(* Logix 5000 Rung export; software revision 24.00 *)

TYPE SNAPP_CONTROL_22 :
STRUCT
   Reserved_0_0 : BOOL;
   Trigger : BOOL;
   Reserved_0_2 : BOOL;
   InspectionResultsAck : BOOL;
   ExecuteCommand : BOOL;
   Reserved_0_5 : BOOL;
   Reserved_0_6 : BOOL;
   Reserved_0_7 : BOOL;
   Reserved_Byte1 : SINT;
   Reserved_2_0 : BOOL;
   Reserved_2_1 : BOOL;
   ClearError : BOOL;
   Reserved_2_3 : BOOL;
   Reserved_2_4 : BOOL;
   Reserved_2_5 : BOOL;
   Reserved_2_6 : BOOL;
   Reserved_2_7 : BOOL;
   Reserved_3_0 : BOOL;
   Reserved_3_1 : BOOL;
   Reserved_3_2 : BOOL;
   Reserved_3_3 : BOOL;
   Reserved_3_4 : BOOL;
   Reserved_3_5 : BOOL;
   Reserved_3_6 : BOOL;
   Reserved_3_7 : BOOL;
   CommandID : INT;
   Reserved_Bytes6and7 : INT;
END_STRUCT
END_TYPE

TYPE SNAPP_IN_13 :
STRUCT
   Status : SNAPP_STAT_IN_13;
   InspectionResults : SNAPP_RESULTS_13;
END_STRUCT
END_TYPE

TYPE SNAPP_STAT_IN_13 :
STRUCT
   TriggerReady : BOOL;
   TriggerAck : BOOL;
   Reserved_0_2 : BOOL;
   AcqError : BOOL;
   Reserved_0_4 : BOOL;
   Reserved_0_5 : BOOL;
   Reserved_0_6 : BOOL;
   Online : BOOL;
   Reserved_1_0 : BOOL;
   InspectionCompleted : BOOL;
   Reserved_1_2 : BOOL;
   ResultsValid : BOOL;
   CommandExecuting : BOOL;
   CommandCompleted : BOOL;
   CommandFailed : BOOL;
   Error : BOOL;
   Reserved_2_0 : BOOL;
   Reserved_2_1 : BOOL;
   Reserved_2_2 : BOOL;
   Reserved_2_3 : BOOL;
   InspectionPass : BOOL;
   Reserved_2_5 : BOOL;
   Reserved_2_6 : BOOL;
   Reserved_2_7 : BOOL;
   Reserved_3_0 : BOOL;
   Reserved_3_1 : BOOL;
   Reserved_3_2 : BOOL;
   Reserved_3_3 : BOOL;
   Reserved_3_4 : BOOL;
   Reserved_3_5 : BOOL;
   Reserved_3_6 : BOOL;
   Reserved_3_7 : BOOL;
   ErrorID : INT;
   Reserved_Bytes_6_7 : INT;
   CurrentProgramID : INT;
   AcquisitionID : INT;
   InspectionID : INT;
   Reserved_Bytes_14_15 : INT;
END_STRUCT
END_TYPE

TYPE SNAPP_RESULTS_13 :   // Inspection Results from Sensor
STRUCT
   PayloadVersion : SINT;
   ApplicationType : SINT;
   Program : SINT;
   InspectionStatusCode : SINT;   // 0=Inspection Valid, 1=Sensor Untrained, 2=Fixture Not Found, 3=ROI Outside Image, 4...255=Reserved
   IdentifiedClassEnum : SINT;   // Anomaly: 0=Reserved, 1=OK, 2=NG, 3-254=Reserved, 255=Error
   IdentifiedClassConfidence : SINT;
   ClassName : SINT[474];
END_STRUCT
END_TYPE

TYPE SNAPP_OUT_22 :
STRUCT
   Control : SNAPP_CONTROL_22;
END_STRUCT
END_TYPE

VAR_GLOBAL   (* controller tags *)
   SNAPP2800_Out : SNAPP_OUT_22 := (Control.CommandID := 1);
   ProgChangeErrorID : INT;
   NewProgramID : INT := 1;
   SNAPPClearError : BOOL;
   SNAPP2800_In : SNAPP_IN_13;
   SNAPPChangeProgram : BOOL;
END_VAR

PROGRAM MainProgram

ROUTINE SNAPPky   (* ladder *)
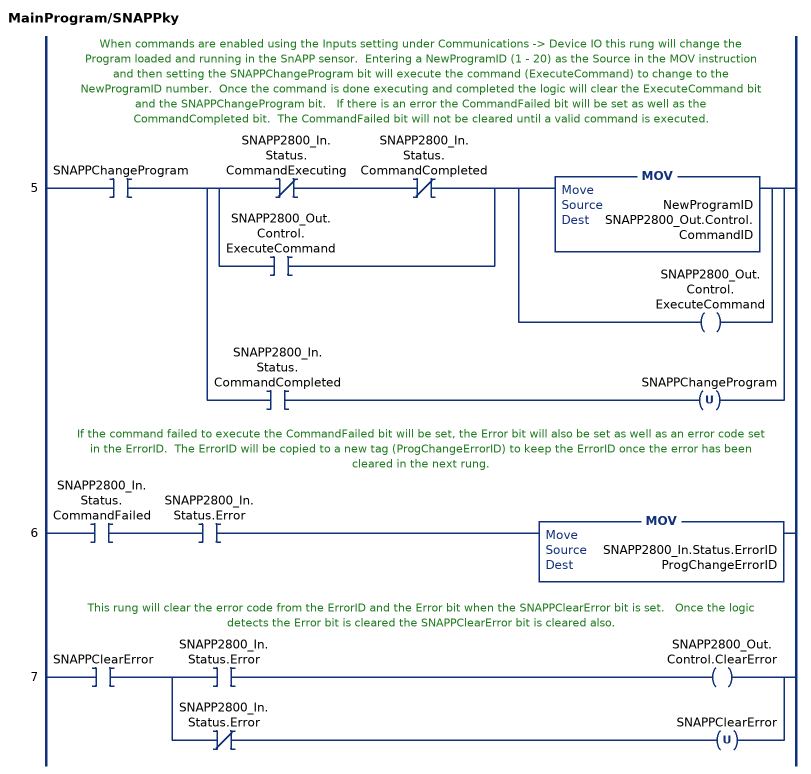
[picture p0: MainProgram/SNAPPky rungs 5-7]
   // When commands are enabled using the Inputs setting under Communications -> Device IO this rung will change the Program loaded and running in the SnAPP sensor.  Entering a NewProgramID (1 - 20) as the Source in the MOV instruction and then setting the SNAPPChangeProgram bit will execute the command (ExecuteCommand) to change to the NewProgramID number.  Once the command is done executing and completed the logic will clear the ExecuteCommand bit and the SNAPPChangeProgram bit.   If there is an error the CommandFailed bit will be set as well as the CommandCompleted bit.  The CommandFailed bit will not be cleared until a valid command is executed.
   5: XIC(SNAPPChangeProgram)[[XIO(SNAPP2800_In.Status.CommandExecuting) XIO(SNAPP2800_In.Status.CommandCompleted) ,XIC(SNAPP2800_Out.Control.ExecuteCommand) ] [MOV(NewProgramID,SNAPP2800_Out.Control.CommandID) ,OTE(SNAPP2800_Out.Control.ExecuteCommand) ] ,XIC(SNAPP2800_In.Status.CommandCompleted) OTU(SNAPPChangeProgram) ];
   // If the command failed to execute the CommandFailed bit will be set, the Error bit will also be set as well as an error code set in the ErrorID.  The ErrorID will be copied to a new tag (ProgChangeErrorID) to keep the ErrorID once the error has been cleared in the next rung.
   6: XIC(SNAPP2800_In.Status.CommandFailed)XIC(SNAPP2800_In.Status.Error)MOV(SNAPP2800_In.Status.ErrorID,ProgChangeErrorID);
   // This rung will clear the error code from the ErrorID and the Error bit when the SNAPPClearError bit is set.   Once the logic detects the Error bit is cleared the SNAPPClearError bit is cleared also.
   7: XIC(SNAPPClearError)[XIC(SNAPP2800_In.Status.Error) OTE(SNAPP2800_Out.Control.ClearError) ,XIO(SNAPP2800_In.Status.Error) OTU(SNAPPClearError) ];
END_ROUTINE
END_PROGRAM
